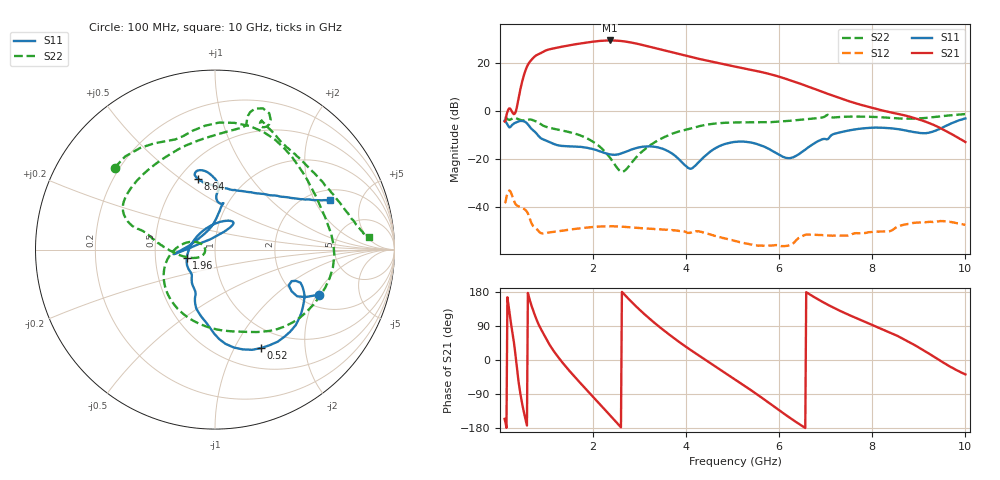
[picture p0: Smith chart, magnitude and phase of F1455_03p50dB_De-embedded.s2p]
! Integrated Device Technology
! Corporate Headquarters
! 6024 Silver Creek Valley Road
! San Jose, CA 95138  USA
! Phone:  1-408-284-8200
! Toll Free:  1-800-223-1366
! Webpage:  http://www.idt.com/
! Timing and RF Division
! 515 Groton Road, Suite 102
! Westford, MA 01886-6024
! Device:  F1455
! Description: 6-bit 0.5 dB Transmit Variable Gain Amplifier
! Frequency:  1400.0 -  2300.00 MHz
! Package:  6x6 mm Thin QFN Plastic Package: 28 pin
! State:  7
! Atten State:  3.5 dB
! Voltage:  +5.00 Volts
! Current:  215.376 mA
! Data:  The device was measured on a the F1455 evaluation board which has
!  individual transmission lines to the RF pins.  Data was collected
!  using a calibrated network analyzer.  The evaluation board was
!  de-embedded using a TRL calibration technique.
!  The reference plane is the edge of the package pin.
!  Pin  1 = CSb
!  Pin  2 = DATA
!  Pin  3 = CLK
!  Pin  4 = RSET
!  Pin  5 = GND
!  Pin  6 = RFIN  = Port 1
!  Pin  7 = GND
!  Pin  8 = NC
!  Pin  9 = NC
!  Pin 10 = NC
!  Pin 11 = NC
!  Pin 12 = NC
!  Pin 13 = NC
!  Pin 14 = /STBY
!  Pin 15 = GND
!  Pin 16 = RFOUT  = Port 2
!  Pin 17 = GND
!  Pin 18 = NC
!  Pin 19 = NC
!  Pin 20 = NC
!  Pin 21 = GND
!  Pin 22 = NC
!  Pin 23 = GND
!  Pin 24 = NC
!  Pin 25 = NC
!  Pin 26 = NC
!  Pin 27 = GND
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# GHz S dB R 50
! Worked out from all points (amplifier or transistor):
!   496 points, 100 MHz to 10 GHz, reference 50 ohm
!   highest |S21| = 29.3 dB at 2.36 GHz (marker M1)
!   |S21| within 3 dB of that: 1.225 GHz to 3.297 GHz (2.072 GHz wide, 91.6 % of centre)
!   unconditionally stable (mu >= 1): start of sweep to end of sweep
!   at 1.74 GHz: K = 4.72, MAG = 28.7 dB, |S12| = -48.7 dB
!   at 5.06 GHz: K = 19.14, MAG = 20.4 dB, |S12| = -54.0 dB
!   at 10 GHz: K = 66.63, MAG = -4.1 dB, |S12| = -47.3 dB
!   S11 on the Smith chart (normalised r, x): 100 MHz: 2.50, -2.10; 520 MHz: 0.74, -1.29; 1.96 GHz: 0.72, -0.07; 8.64 GHz: 0.62, +0.58; 10 GHz: 2.50, +2.72
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0.1  -3.98 -23.5  -4.39 -155.5  -38.18 40.6  -2.83 140.8
0.38  -4.48 -36.4  3.13 -37.8  -39.42 -107.3  -3.29 55.9
0.52  -4.35 -64.8  15.18 -140.9  -40.71 -151.6  -3.95 24.3
0.7  -7.82 -97.3  21.73 135.4  -47.42 152.1  -3.75 -19.3
0.82  -10.20 -111.2  23.50 96.7  -49.70 135.2  -4.77 -47.9
0.96  -12.07 -117.2  24.90 63.5  -50.77 124.8  -6.37 -72.2
1.14  -13.57 -128.5  25.93 26.4  -50.22 102.7  -7.32 -96.8
1.34  -14.50 -134.3  26.72 -6.3  -49.70 81.3  -8.12 -120.4
1.76  -14.96 -150.4  28.13 -65.2  -48.60 46.4  -10.40 -159.4
1.96  -15.65 -162.8  28.68 -91.7  -48.25 32.7  -12.29 -175.7
2.16  -16.86 178.2  29.10 -118.3  -47.97 19.7  -15.09 168.8
2.36  -18.03 149.2  29.27 -145.3  -47.88 7.1  -19.30 157.7
2.62  -17.57 104.0  29.01 179.9  -48.04 -8.2  -25.28 -178.7
2.92  -15.47 71.1  28.03 142.0  -48.50 -22.8  -19.41 -155.7
3.4  -15.15 54.5  25.77 90.0  -49.11 -42.3  -12.18 -178.3
4.06  -23.83 105.6  22.58 29.5  -50.64 -67.5  -7.45 165.4
5.06  -12.79 -173.8  18.40 -52.0  -54.02 -104.7  -4.76 148.9
5.92  -17.34 167.5  14.68 -125.6  -55.69 -110.7  -4.51 110.3
6.7  -14.11 85.1  9.57 169.8  -51.32 -137.9  -3.20 78.4
8.36  -7.13 104.6  -0.48 73.3  -49.97 168.0  -2.83 62.4
8.64  -7.83 103.6  -1.59 57.2  -47.39 161.3  -3.16 53.4
10  -3.09 23.3  -12.91 -38.0  -47.30 83.0  -1.29 4.6
